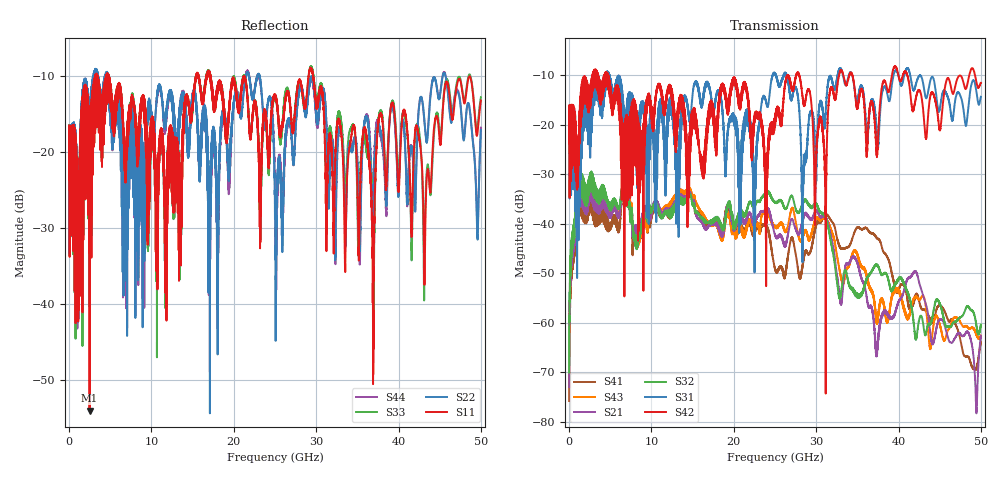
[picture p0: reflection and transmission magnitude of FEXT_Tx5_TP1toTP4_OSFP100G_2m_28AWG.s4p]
! Touchstone data
! Created: 27-Feb-2019 by IdEM 12 (12.1.0)
! COMMENTS
!  Created Wed Feb 27 12:03:36 2019
!  64 Port Network Data from SP1.SP block
!  freq  magS1_1  angS1_1  magS1_2  angS1_2  magS1_3  angS1_3  magS1_4  angS1_4
!  magS1_5  angS1_5  magS1_6  angS1_6  magS1_7  angS1_7  magS1_8  angS1_8
!  magS1_9  angS1_9  magS1_10  angS1_10  magS1_11  angS1_11  magS1_12  angS1_12
!  magS1_13  angS1_13  magS1_14  angS1_14  magS1_15  angS1_15  magS1_16  angS1_16
!  magS1_17  angS1_17  magS1_18  angS1_18  magS1_19  angS1_19  magS1_20  angS1_20
!  magS1_21  angS1_21  magS1_22  angS1_22  magS1_23  angS1_23  magS1_24  angS1_24
!  magS1_25  angS1_25  magS1_26  angS1_26  magS1_27  angS1_27  magS1_28  angS1_28
!  magS1_29  angS1_29  magS1_30  angS1_30  magS1_31  angS1_31  magS1_32  angS1_32
!  magS1_33  angS1_33  magS1_34  angS1_34  magS1_35  angS1_35  magS1_36  angS1_36
!  magS1_37  angS1_37  magS1_38  angS1_38  magS1_39  angS1_39  magS1_40  angS1_40
!  magS1_41  angS1_41  magS1_42  angS1_42  magS1_43  angS1_43  magS1_44  angS1_44
!  magS1_45  angS1_45  magS1_46  angS1_46  magS1_47  angS1_47  magS1_48  angS1_48
!  magS1_49  angS1_49  magS1_50  angS1_50  magS1_51  angS1_51  magS1_52  angS1_52
!  magS1_53  angS1_53  magS1_54  angS1_54  magS1_55  angS1_55  magS1_56  angS1_56
!  magS1_57  angS1_57  magS1_58  angS1_58  magS1_59  angS1_59  magS1_60  angS1_60
!  magS1_61  angS1_61  magS1_62  angS1_62  magS1_63  angS1_63  magS1_64  angS1_64
!  magS2_1  angS2_1  magS2_2  angS2_2  magS2_3  angS2_3  magS2_4  angS2_4
!  magS2_5  angS2_5  magS2_6  angS2_6  magS2_7  angS2_7  magS2_8  angS2_8
!  magS2_9  angS2_9  magS2_10  angS2_10  magS2_11  angS2_11  magS2_12  angS2_12
!  magS2_13  angS2_13  magS2_14  angS2_14  magS2_15  angS2_15  magS2_16  angS2_16
!  magS2_17  angS2_17  magS2_18  angS2_18  magS2_19  angS2_19  magS2_20  angS2_20
!  magS2_21  angS2_21  magS2_22  angS2_22  magS2_23  angS2_23  magS2_24  angS2_24
!  magS2_25  angS2_25  magS2_26  angS2_26  magS2_27  angS2_27  magS2_28  angS2_28
!  magS2_29  angS2_29  magS2_30  angS2_30  magS2_31  angS2_31  magS2_32  angS2_32
!  magS2_33  angS2_33  magS2_34  angS2_34  magS2_35  angS2_35  magS2_36  angS2_36
!  magS2_37  angS2_37  magS2_38  angS2_38  magS2_39  angS2_39  magS2_40  angS2_40
!  magS2_41  angS2_41  magS2_42  angS2_42  magS2_43  angS2_43  magS2_44  angS2_44
!  magS2_45  angS2_45  magS2_46  angS2_46  magS2_47  angS2_47  magS2_48  angS2_48
!  magS2_49  angS2_49  magS2_50  angS2_50  magS2_51  angS2_51  magS2_52  angS2_52
!  magS2_53  angS2_53  magS2_54  angS2_54  magS2_55  angS2_55  magS2_56  angS2_56
!  magS2_57  angS2_57  magS2_58  angS2_58  magS2_59  angS2_59  magS2_60  angS2_60
!  magS2_61  angS2_61  magS2_62  angS2_62  magS2_63  angS2_63  magS2_64  angS2_64
!  magS3_1  angS3_1  magS3_2  angS3_2  magS3_3  angS3_3  magS3_4  angS3_4
!  magS3_5  angS3_5  magS3_6  angS3_6  magS3_7  angS3_7  magS3_8  angS3_8
!  magS3_9  angS3_9  magS3_10  angS3_10  magS3_11  angS3_11  magS3_12  angS3_12
!  magS3_13  angS3_13  magS3_14  angS3_14  magS3_15  angS3_15  magS3_16  angS3_16
!  magS3_17  angS3_17  magS3_18  angS3_18  magS3_19  angS3_19  magS3_20  angS3_20
!  magS3_21  angS3_21  magS3_22  angS3_22  magS3_23  angS3_23  magS3_24  angS3_24
!  magS3_25  angS3_25  magS3_26  angS3_26  magS3_27  angS3_27  magS3_28  angS3_28
!  magS3_29  angS3_29  magS3_30  angS3_30  magS3_31  angS3_31  magS3_32  angS3_32
!  magS3_33  angS3_33  magS3_34  angS3_34  magS3_35  angS3_35  magS3_36  angS3_36
!  magS3_37  angS3_37  magS3_38  angS3_38  magS3_39  angS3_39  magS3_40  angS3_40
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# Hz S MA R 50
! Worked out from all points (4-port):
!   5000 points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, 10 MHz to 50 GHz, reference 50 ohm
!   strongest paths, dB at 10 MHz, 12.51 GHz, 25.01 GHz, 37.51 GHz, 50 GHz:
!     S42: -18.0, -13.7, -18.1, -22.5, -11.5
!     S31: -18.0, -16.4, -9.6, -24.1, -14.3
!     S32: -70.1, -38.0, -35.6, -48.6, -60.4
!     S21: -73.0, -37.4, -42.3, -64.2, -62.6
!     S43: -72.9, -36.0, -40.5, -59.3, -62.6
!     S41: -75.8, -37.1, -49.2, -43.1, -63.9
!   lowest |S11| = -54.1 dB at 2.49 GHz (marker M1), VSWR 1.00, Z = 49.8 + j0.0446 ohm
!   |S11| at or under -10 dB: 4.81 GHz to 15.41 GHz (10.6 GHz wide, 105 % of centre); 17.19 GHz to 29.09 GHz (11.9 GHz wide, 51.4 % of centre); 29.64 GHz to end of sweep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
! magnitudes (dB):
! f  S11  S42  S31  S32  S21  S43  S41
! 10 MHz  -17.7  -18.0  -18.0  -70.1  -73.0  -72.9  -75.8
! 2.49 GHz  -54.1  -16.3  -22.3  -33.3  -35.3  -34.8  -37.1
! 23.93 GHz  -15.4  -52.6  -15.4  -33.7  -37.1  -37.8  -40.5
! 26.54 GHz  -12.0  -10.1  -11.0  -36.3  -42.5  -40.7  -47.1
! 28.46 GHz  -13.3  -15.5  -30.1  -35.7  -38.9  -42.3  -47.4
! 32.9 GHz  -16.3  -9.3  -8.6  -55.0  -55.3  -50.0  -44.6
! 50 GHz  -13.3  -11.5  -14.3  -60.4  -62.6  -62.6  -63.9
